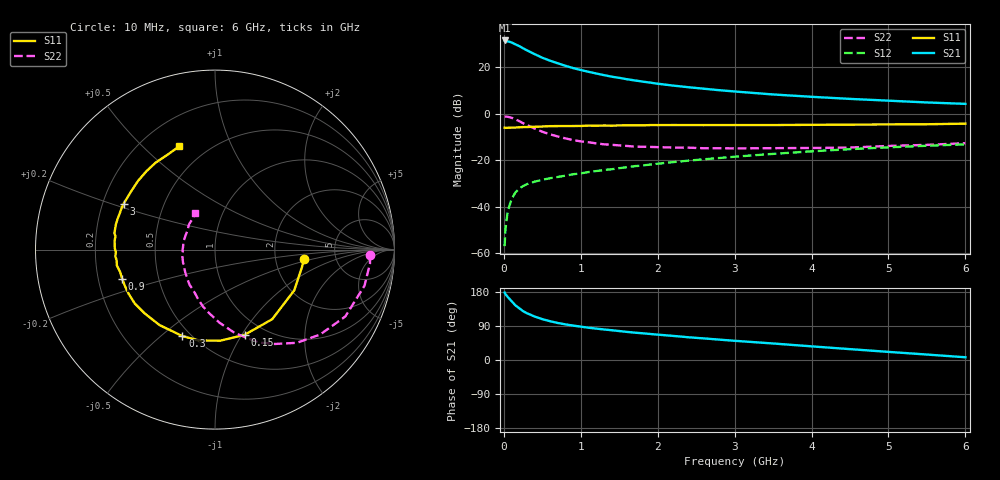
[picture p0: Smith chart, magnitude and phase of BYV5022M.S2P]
! SIEMENS Small Signal Semiconductors
! BFY420
! Si NPN RF SIEGET Grounded Emitter Transistor in MICRO-X
! VCE = 0.5 V  IC = 22 mA
! Common Emitter S-Parameters:  October  1996
# GHz  S  MA  R  50
!  f  S11  S21  S12  S22
! GHz  MAG  ANG  MAG  ANG  MAG  ANG  MAG  ANG
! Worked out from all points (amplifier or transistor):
!   36 points, 10 MHz to 6 GHz, reference 50 ohm
!   highest |S21| = 31.5 dB at 10 MHz (marker M1)
!   |S21| within 3 dB of that: start of sweep to 230.2 MHz
!   unconditionally stable (mu >= 1): start of sweep to 16.26 MHz; 1.341 GHz to end of sweep
!   at 250 MHz: K = 0.37, MSG = 29.7 dB, |S12| = -31.2 dB
!   at 1.4 GHz: K = 1.03, MAG = 19.0 dB, |S12| = -24.0 dB
!   at 6 GHz: K = 1.14, MAG = 6.4 dB, |S12| = -13.2 dB
!   S11 on the Smith chart (normalised r, x): 10 MHz: 2.92, -0.41; 150 MHz: 0.81, -1.03; 300 MHz: 0.45, -0.59; 900 MHz: 0.30, -0.14; 3 GHz: 0.29, +0.22; 6 GHz: 0.36, +0.65
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0.01  0.4976 -6.1  37.74 178.0  0.0014 97.8  0.8641 -2.1
0.02  0.4941 -11.6  37.5 174.1  0.0032 85.0  0.867 -5.1
0.05  0.4965 -27.2  36.14 166.5  0.0078 79.1  0.8571 -13.6
0.1  0.502 -50.6  34.27 155.4  0.0145 71.2  0.816 -27.2
0.15  0.5026 -70.9  31.18 144.2  0.02 64.7  0.7532 -38.9
0.2  0.5082 -86.5  28.52 136.6  0.0242 59.4  0.6912 -48.7
0.25  0.5142 -100.2  25.59 128.9  0.0276 55.9  0.6228 -57.6
0.3  0.515 -110.6  23.14 123.4  0.0303 53.3  0.5713 -64.9
0.4  0.5219 -126.3  19.18 114.8  0.0343 49.4  0.4781 -76.6
0.5  0.529 -137.8  16.02 107.8  0.0376 47.7  0.4086 -86.4
0.6  0.5386 -146.2  13.84 102.4  0.0407 47.0  0.3589 -94.6
0.7  0.5403 -152.8  12.18 97.7  0.0433 47.2  0.3231 -102.1
0.9  0.5421 -162.7  9.605 90.8  0.0496 48.1  0.269 -114.2
1.1  0.5537 -170.7  7.976 85.2  0.0553 49.0  0.2424 -125.6
1.4  0.5523 -178.7  6.27 78.6  0.0634 49.5  0.2138 -139.4
1.6  0.5603 176.6  5.511 74.2  0.0703 49.3  0.2017 -147.4
2.2  0.5698 165.5  4.025 63.6  0.0904 47.9  0.1864 -165.7
3  0.5694 153.2  3.005 50.7  0.1183 43.4  0.1787 175.4
3.5  0.5688 145.6  2.593 43.6  0.1361 39.8  0.1808 165.7
4.5  0.5803 131.1  2.081 28.7  0.1719 30.3  0.1863 145.3
5.5  0.5919 116.0  1.743 14.4  0.2039 19.8  0.2128 125.9
6  0.6092 109.1  1.626 7.2  0.2183 14.4  0.2312 118.2
